(* SV ASDU data type (TwinCAT PLC little endian host byte order) *)
TYPE ST_SVASDU_IED_MUnn_LLN0_MSVCB01 : 
STRUCT
	nSmpCnt: UINT; (* Sample counter *)
	eSmpSynch: E_GseSvSmpSynch; (* Synchronization type: 0..2 *)
	tRefrTm: T_UtcTime; (* Sample refresh time stamp (optional) *)
	
	IED_MUnn_InnATCTR1_AmpSv_instMag_i: DINT;
	IED_MUnn_InnATCTR1_AmpSv_q: ST_AcsiQuality;
	IED_MUnn_InnBTCTR2_AmpSv_instMag_i: DINT;
	IED_MUnn_InnBTCTR2_AmpSv_q: ST_AcsiQuality;
	IED_MUnn_InnCTCTR3_AmpSv_instMag_i: DINT;
	IED_MUnn_InnCTCTR3_AmpSv_q: ST_AcsiQuality;
	IED_MUnn_InnNTCTR4_AmpSv_instMag_i: DINT;
	IED_MUnn_InnNTCTR4_AmpSv_q: ST_AcsiQuality;
	IED_MUnn_UnnATVTR1_VolSv_instMag_i: DINT;
	IED_MUnn_UnnATVTR1_VolSv_q: ST_AcsiQuality;
	IED_MUnn_UnnBTVTR2_VolSv_instMag_i: DINT;
	IED_MUnn_UnnBTVTR2_VolSv_q: ST_AcsiQuality;
	IED_MUnn_UnnCTVTR3_VolSv_instMag_i: DINT;
	IED_MUnn_UnnCTVTR3_VolSv_q: ST_AcsiQuality;
	IED_MUnn_UnnNTVTR4_VolSv_instMag_i: DINT;
	IED_MUnn_UnnNTVTR4_VolSv_q: ST_AcsiQuality;
END_STRUCT
END_TYPE
